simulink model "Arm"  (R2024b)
settings: Solver=VariableStepAuto  StartTime=0.0  StopTime=10.0  RelTol=1e-3
undefined symbols (not defined in the file): deg, kg, m, N, s, X, Y, Z
libraries: sm_lib x7, nesl_utility x1

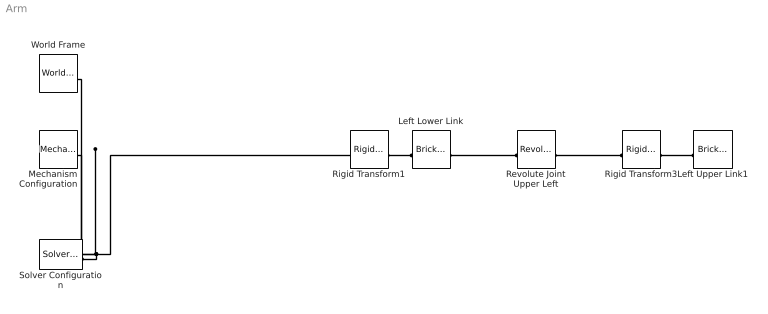
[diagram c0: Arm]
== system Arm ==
  Left Lower Link : sm_lib/Body Elements/Brick Solid  BrickDimensions=[2 12 0.5]  BrickDimensionsUnits=cm  ExportEntireGeometry=off  InertiaType=CalculateFromGeometry  BasedOnType=Density  Density=1000  DensityUnits=kg/m^3  Mass=1  MassUnits=kg  CenterOfMass=[0 0 0]  CenterOfMassUnits=m  MomentsOfInertia=[1 1 1]  MomentsOfInertiaUnits=kg*m^2  ProductsOfInertia=[0 0 0]  ProductsOfInertiaUnits=kg*m^2  GraphicType=FromGeometry  MarkerShape=Sphere  MarkerSize=10  GraphicVisPropType=SimpleVisualProperties  GraphicDiffuseColor=[0.5 0.5 0.5]  GraphicOpacity=1  GraphicSpecularColor=[0.5 0.5 0.5 1.0]  GraphicAmbientColor=[0.15 0.15 0.15 1.0]  GraphicEmissiveColor=[0.0 0.0 0.0 1.0]  GraphicShininess=75  DoExposeReferenceFrame=on  SerializedFrames=<Frames><Frame><Id>Frame1</Id><Value><Name>F1</Name><Origin><Source>ReferenceFrame</Source><FeatureName></FeatureName></Origin><PrimaryAxis><DefinedDirection>+Z</DefinedDirection><Source>ReferenceFrame</Source><SourceDirection>+Z</SourceDirection><FeatureName></FeatureName></PrimaryAxis><SecondaryAxis><DefinedDirection>+X</DefinedDirection><Source>ReferenceFrame</Source><SourceDirection>+X</Source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
  Left Upper Link1 : sm_lib/Body Elements/Brick Solid  BrickDimensions=[2 12 0.5]  BrickDimensionsUnits=cm  ExportEntireGeometry=off  InertiaType=CalculateFromGeometry  BasedOnType=Density  Density=1000  DensityUnits=kg/m^3  Mass=1  MassUnits=kg  CenterOfMass=[0 0 0]  CenterOfMassUnits=m  MomentsOfInertia=[1 1 1]  MomentsOfInertiaUnits=kg*m^2  ProductsOfInertia=[0 0 0]  ProductsOfInertiaUnits=kg*m^2  GraphicType=FromGeometry  MarkerShape=Sphere  MarkerSize=10  GraphicVisPropType=SimpleVisualProperties  GraphicDiffuseColor=[0.5 0.5 0.5]  GraphicOpacity=1  GraphicSpecularColor=[0.5 0.5 0.5 1.0]  GraphicAmbientColor=[0.15 0.15 0.15 1.0]  GraphicEmissiveColor=[0.0 0.0 0.0 1.0]  GraphicShininess=75  DoExposeReferenceFrame=on  SerializedFrames=<Frames><Frame><Id>Frame1</Id><Value><Name>F1</Name><Origin><Source>ReferenceFrame</Source><FeatureName></FeatureName></Origin><PrimaryAxis><DefinedDirection>+Z</DefinedDirection><Source>ReferenceFrame</Source><SourceDirection>+Z</SourceDirection><FeatureName></FeatureName></PrimaryAxis><SecondaryAxis><DefinedDirection>+X</DefinedDirection><Source>ReferenceFrame</Source><SourceDirection>+X</Source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
  Mechanism Configuration : sm_lib/Utilities/Mechanism Configuration  UniformGravity=Constant  GravityVector=[0 0 -9.80665]  GravityVectorUnits=m/s^2  LinearizationDelta=0.001  JointModeTransitionNonlinearIterations=2
  Revolute Joint Upper Left : sm_lib/Joints/Revolute Joint  JointMode=Normal  CompositeWrenchDir=FollowerOnBase  CompositeWrenchFrame=BaseFrame  SenseConstraintForce=off  SenseConstraintTorque=off  SenseTotalForce=off  SenseTotalTorque=off  PositionTargetSpecify=off  PositionTargetPriority=High  PositionTargetValue=0  PositionTargetValueUnits=deg  VelocityTargetSpecify=off  VelocityTargetPriority=High  VelocityTargetValue=0  VelocityTargetValueUnits=deg/s  EquilibriumPosition=0  EquilibriumPositionUnits=deg  SpringStiffness=0  SpringStiffnessUnits=N*m/deg  DampingCoefficient=0  DampingCoefficientUnits=N*m/(deg/s)  LowerLimitSpecify=off  LowerLimitBound=-90  LowerLimitBoundUnits=deg  LowerLimitStiffness=1e4  LowerLimitStiffnessUnits=N*m/deg  LowerLimitDamping=10  LowerLimitDampingUnits=N*m/(deg/s)  LowerLimitTransitionRegionWidth=0.1  LowerLimitTransitionRegionWidthUnits=deg  UpperLimitSpecify=off  UpperLimitBound=90  UpperLimitBoundUnits=deg  UpperLimitStiffness=1e4  UpperLimitStiffnessUnits=N*m/deg  UpperLimitDamping=10  UpperLimitDampingUnits=N*m/(deg/s)  UpperLimitTransitionRegionWidth=0.1  UpperLimitTransitionRegionWidthUnits=deg  TorqueActuationMode=NoTorque  MotionActuationMode=ComputedMotion  SensePosition=off  SenseVelocity=off  SenseAcceleration=off  SenseTorqueForce=off  SenseLowerLimitTorqueForce=off  SenseUpperLimitTorqueForce=off
  Rigid Transform1 : sm_lib/Frames and Transforms/Rigid Transform  RotationMethod=StandardAxis  FollAlignAxisA=+X  BaseAlignAxisA=+Y  FollAlignAxisB=+Y  BaseAlignAxisB=+Z  RotationStandardAxis=+Z  RotationAngle=30  RotationAngleUnits=deg  RotationArbitraryAxis=[0 0 1]  RotationSequenceAxes=FollowerAxes  RotationSequence=XYX  RotationSequenceAngles=[0 0 0]  RotationSequenceAnglesUnits=deg  RotationMatrix=[1 0 0;0 1 0;0 0 1]  Quaternion=[1 0 0 0]  TranslationMethod=Cartesian  TranslationCartesianOffset=[-1 5 3]  TranslationCartesianOffsetUnits=cm  TranslationStandardAxis=+Z  TranslationStandardOffset=0  TranslationStandardOffsetUnits=m  TranslationROffset=0  TranslationROffsetUnits=m  TranslationThetaOffset=0  TranslationThetaOffsetUnits=deg  TranslationZOffset=0  TranslationZOffsetUnits=m
  Rigid Transform3 : sm_lib/Frames and Transforms/Rigid Transform  RotationMethod=StandardAxis  FollAlignAxisA=+X  BaseAlignAxisA=+Y  FollAlignAxisB=+Y  BaseAlignAxisB=+Z  RotationStandardAxis=+Z  RotationAngle=-75  RotationAngleUnits=deg  RotationArbitraryAxis=[0 0 1]  RotationSequenceAxes=FollowerAxes  RotationSequence=XYX  RotationSequenceAngles=[0 0 0]  RotationSequenceAnglesUnits=deg  RotationMatrix=[1 0 0;0 1 0;0 0 1]  Quaternion=[1 0 0 0]  TranslationMethod=Cartesian  TranslationCartesianOffset=[4.8 7 0.6]  TranslationCartesianOffsetUnits=cm  TranslationStandardAxis=+Z  TranslationStandardOffset=0  TranslationStandardOffsetUnits=m  TranslationROffset=0  TranslationROffsetUnits=m  TranslationThetaOffset=0  TranslationThetaOffsetUnits=deg  TranslationZOffset=0  TranslationZOffsetUnits=m
  Solver Configuration : nesl_utility/Solver Configuration  PhysicalDomain=network_engine_domain  SubClassName=solver  LeftPortType=input  RightPortType=generic  Tones=[]  Harmonics=[]  SimulateNoise=off  Profile=off  UseLocalSampling=off  EnableSwitchedLinearOptims=on  FrequencyDomain=off  UseCCode=off  RelTol=0.001  AbsTol=0.001  MinStep=1e-09  ToWorkspace=off  RevertToSquareIcSolve=off  NumHomotopyIterations=100  PhasorMode=off  PhasorModeNumHarmonics=1  ConsistencySolver=NEWTON_XTOL_AFTER_FTOL  IndexReductionMethod=DerivativeReplacement  DoDC=off  ResidualTolerance=1e-09  ConsistencyTolSource=GLOBAL  ConsistencyAbsTol=0.001  ConsistencyRelTol=0.001  ConsistencyTolFactor=0.001  UseLocalSolver=off  LocalSolverChoice=NE_BACKWARD_EULER_ADVANCER  ResolveIndetEquations=on  FunctionEvalNumThread=1  LocalSolverSampleTime=0.001  DoFixedCost=off  MaxNonlinIter=3  MaxModeIter=2  ComputeImpulses=off  ImpulseIterations=2  LinearAlgebra=auto  LinearAlgebraNumThread=0  EquationFormulation=NE_TIME_EF  DelaysMemoryBudget=1024  AutomaticFiltering=on  FilteringTimeConstant=0.001  PartitionStorageMethod=AS_NEEDED  PartitionMemoryBudget=1024  PartitionMethod=ROBUST  MultibodyUseLocalSolver=off  MultibodyLocalSolverChoice=ODE1  MultibodyLocalSolverSampleTime=0.001
  World Frame : sm_lib/Frames and Transforms/World Frame
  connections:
  Revolute Joint Upper Left/LConn1 -- Left Lower Link/RConn1
  Rigid Transform1/RConn1 -- Left Lower Link/LConn1
  Rigid Transform3/RConn1 -- Left Upper Link1/LConn1
  Revolute Joint Upper Left/RConn1 -- Rigid Transform3/LConn1
  Solver Configuration/RConn1 -- World Frame/RConn1 -- Rigid Transform1/LConn1 -- Mechanism Configuration/RConn1
